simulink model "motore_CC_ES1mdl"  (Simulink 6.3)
settings: Solver=ode45  StartTime=0.0  StopTime=10.0  RelTol=1e-6  AbsTol=1e-6
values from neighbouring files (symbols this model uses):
  b = k*(T-2*tau1)    (= -1.462)    [Formule_di_Inversione_discrete.m]    (also in Esempio0.m = 0.1; Controllo_CC_K.m = 0.008; motore_CC_ES1.m = 0.8)
  Imax = 10000*Amp    (= 10000)    [Controllo_CC_K.m]    (also in motore_CC_ES1.m = 5)
  J = 0.030*kg*m^2    (= 0.03)    [Controllo_CC_K.m]    (also in motore_CC_ES1.m = 1.6)
  Ke = 0.5*N*m/Amp    (= 0.5)    [Controllo_CC_K.m]    (also in motore_CC_ES1.m = 8)
  L = 0.01*Henry    (= 0.01)    [Controllo_CC_K.m]    (also in motore_CC_ES1.m = 0.1)
  R = 1*Ohm    (= 1)    [Controllo_CC_K.m]    (also in motore_CC_ES1.m = 8)
libraries: slctrlobsolete x3

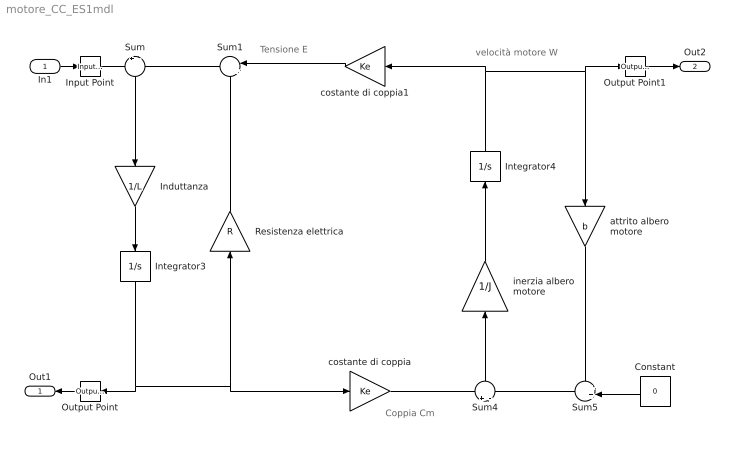
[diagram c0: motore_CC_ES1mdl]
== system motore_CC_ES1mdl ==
  note: Tensione E
  note: velocità motore W
  note: Coppia Cm
  In1 : Inport
  Constant : Constant  Orientation=left  Value=0
  Induttanza : Gain  Orientation=down  Gain=1/L
  Input Point : slctrlobsolete/Input Point
  Integrator3 : Integrator  Orientation=down  LimitOutput=on  UpperSaturationLimit=Imax  LowerSaturationLimit=-Imax
  Integrator4 : Integrator  Orientation=up
  Output Point : slctrlobsolete/Output Point  Orientation=left
  Output Point1 : slctrlobsolete/Output Point
  Resistenza elettrica : Gain  Orientation=up  Gain=R
  Sum : Sum  Orientation=down  Inputs=+|-
  Sum1 : Sum  Orientation=left  Inputs=|++
  Sum4 : Sum  Orientation=up  Inputs=+|-
  Sum5 : Sum  Orientation=left  Inputs=++|
  attrito albero motore : Gain  Orientation=down  Gain=b
  costante di coppia : Gain  Gain=Ke
  costante di coppia1 : Gain  Orientation=left  Gain=Ke
  inerzia albero motore : Gain  Orientation=up  Gain=1/J
  Out1 : Outport  Orientation=left
  Out2 : Outport  Port=2
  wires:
  Sum/1 -> Induttanza/1
  Induttanza/1 -> Integrator3/1
  Sum1/1 -> Sum/2
  Resistenza elettrica/1 -> Sum1/2
  Sum4/1 -> inerzia albero motore/1
  inerzia albero motore/1 -> Integrator4/1
  Sum5/1 -> Sum4/2
  attrito albero motore/1 -> Sum5/1
  Integrator4/1 -> costante di coppia1/1, attrito albero motore/1, Output Point1/1
  costante di coppia1/1 -> Sum1/1
  Constant/1 -> Sum5/2
  costante di coppia/1 -> Sum4/1
  Integrator3/1 -> Resistenza elettrica/1, costante di coppia/1, Output Point/1
  In1/1 -> Input Point/1
  Input Point/1 -> Sum/1
  Output Point/1 -> Out1/1
  Output Point1/1 -> Out2/1
